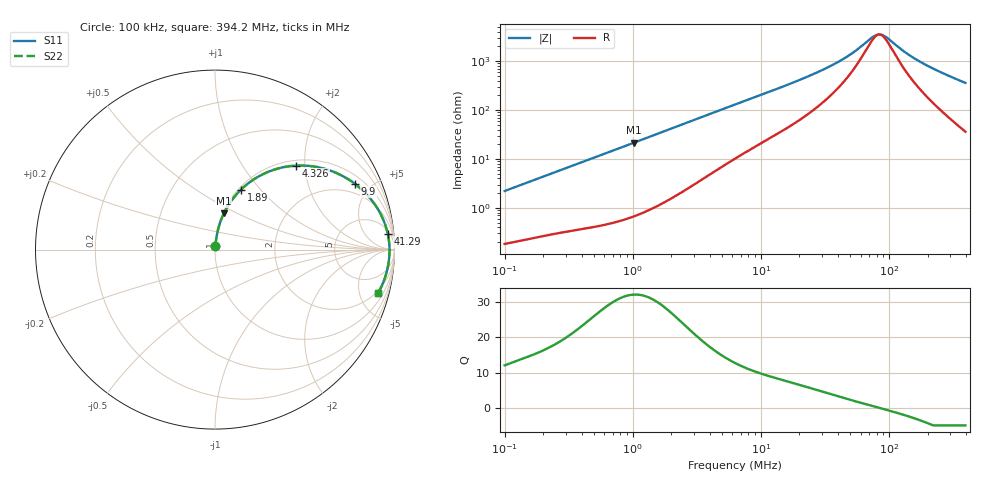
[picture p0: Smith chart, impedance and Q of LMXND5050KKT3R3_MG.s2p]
! LMXND5050KKT3R3_MG  S-PARAMETER MODEL  ( General Type )
! Model Generated by TAIYO YUDEN Corporation (http://www.ty-top.com)
! Version 1.0
! TAIYO YUDEN Control No. 191023NI43SB-FBB
! Copyright(c) 2019 TAIYO YUDEN CO.,LTD. All Rights Reserved.
! Product Description (link to TY-COMPAS)
! https://ds.yuden.co.jp/TYCOMPAS/or/detail?pn=LMXND5050KKT3R3MMG&u=M
! Products Name : Inductors
! Characteristics :
!  Inductance : 3.3 uH , SRF(min) : 42 MHz , DC Resistance(max) : 0.15 Ohm
!  Rated Current : Saturation :1400 mA , Temp Rise : 1250 mA
!  Case Size : 4.9 x 4.9 / 0.193 x 0.193 [mm/inch] , Thickness : 1 / 0.039 [mm/inch]
!  (Conditions: Temperature = 25 degC , DC Bias Current/Voltage = 0A / 0V)
! External Node Assignments :
!  1  o---GGG---o  2
! GND o---------o GND
! Frequency Range : 0.1MHz  -  394.189695MHz  [ 402 STEP ]
# MHz S RI R 50
! Freq[MHz].  S11 Real  S11 Imag  S21 Real  S21 Imag  S12 Real  S12 Imag  S22 Real  S22 Imag
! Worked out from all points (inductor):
!   401 points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, 100 kHz to 394.2 MHz, reference 50 ohm
!   read as one part in series: L = 3.49 uH near 104.2 kHz
!   highest Q = 32.1 at 1.016 MHz (marker M1), where L = 3.36 uH
!   self-resonance near 83.85 MHz
!   S11 on the Smith chart (normalised r, x): 100 kHz: 1.00, +0.04; 1.89 MHz: 1.03, +0.79; 4.326 MHz: 1.11, +1.80; 9.9 MHz: 1.41, +4.02; 41.29 MHz: 7, +19; 394.2 MHz: 1.72, -7.16
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0.1  0.00231 0.022  0.9977 -0.022  0.9977 -0.022  0.00231 0.022
0.400203  0.0108 0.084  0.9892 -0.084  0.9892 -0.084  0.0108 0.084
1.015775  0.0497 0.2023  0.9503 -0.2023  0.9503 -0.2023  0.0497 0.2023
1.601627  0.1101 0.2966  0.8899 -0.2966  0.8899 -0.2966  0.1101 0.2966
1.890059  0.1453 0.3348  0.8547 -0.3348  0.8547 -0.3348  0.1453 0.3348
2.743356  0.258 0.4157  0.742 -0.4157  0.742 -0.4157  0.258 0.4157
4.325595  0.4509 0.4679  0.5491 -0.4679  0.5491 -0.4679  0.4509 0.4679
6.278453  0.6178 0.4482  0.3822 -0.4482  0.3822 -0.4482  0.6178 0.4482
9.899572  0.7803 0.3661  0.2197 -0.3661  0.2197 -0.3661  0.7803 0.3661
15.28942  0.8783 0.2686  0.1217 -0.2686  0.1217 -0.2686  0.8783 0.2686
25.12657  0.9372 0.1677  0.0628 -0.1677  0.0628 -0.1677  0.9372 0.1677
41.29292  0.9626 0.0881  0.0374 -0.0881  0.0374 -0.0881  0.9626 0.0881
52.93547  0.9684 0.0551  0.0316 -0.0551  0.0316 -0.0551  0.9684 0.0551
72.20806  0.9719 0.0174  0.0281 -0.0174  0.0281 -0.0174  0.9719 0.0174
78.44093  0.9722 0.00776  0.0278 -0.00776  0.0278 -0.00776  0.9722 0.00776
86.99395  0.9724 -0.00429  0.0276 0.00429  0.0276 0.00429  0.9724 -0.00429
92.56714  0.9723 -0.0115  0.0277 0.0115  0.0277 0.0115  0.9723 -0.0115
100.5574  0.9721 -0.0213  0.0279 0.0213  0.0279 0.0213  0.9721 -0.0213
134.358  0.9694 -0.0568  0.0306 0.0568  0.0306 0.0568  0.9694 -0.0568
175.8426  0.9637 -0.0936  0.0363 0.0936  0.0363 0.0936  0.9637 -0.0936
260.5674  0.9465 -0.1581  0.0535 0.1581  0.0535 0.1581  0.9465 -0.1581
394.1897  0.9072 -0.2441  0.0928 0.2441  0.0928 0.2441  0.9072 -0.2441
